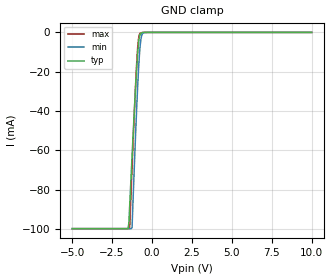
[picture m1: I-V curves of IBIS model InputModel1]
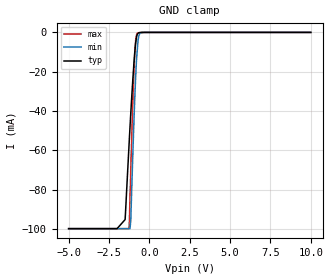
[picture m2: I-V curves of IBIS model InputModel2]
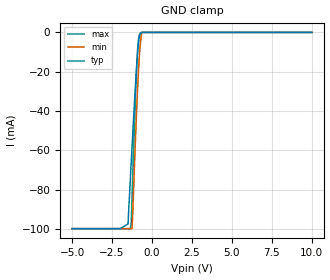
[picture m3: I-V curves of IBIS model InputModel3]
[IBIS Ver]   2.1
[File name]   e_200bx5.ibs   | e_= TSOP, f200bx= abbr chip name, 5= 5V Vcc
[File Rev]   2.00
[Date]   14-February-96
[Source]   File generated from lab measurements at Intel Corporation
[Notes]   Rev 2.00 All data was replaced by actual measurements
   performed in a lab.
[Disclaimer] INTEL DEVELOPER'S SOFTWARE LICENSE AGREEMENT
| BY USING THIS SOFTWARE, YOU ARE AGREEING TO BE BOUND
| BY THE TERMS OFTHIS AGREEMENT.  DO NOT USE THE SOFTWARE
| UNTIL YOU HAVE CAREFULLY READAND AGREED TO THE FOLLOWING
| TERMS AND CONDITIONS.  IF YOU DO NOT AGREETO THE TERMS
| OF THIS AGREEMENT, PROMPTLY RETURN THE SOFTWARE PACKAGE
| ANDANY ACCOMPANYING ITEMS.
| IF YOU USE THIS SOFTWARE, YOU WILL BE BOUND BY THE TERMS
| OF THIS AGREEMENT
| LICENSE: Intel Corporation ("Intel") grants you the non-exclusive right
| to use the enclosed software program ("Software").  You will not use,
| copy, modify, rent, sell or transfer the Software or any portion
| thereof, except as provided in this Agreement.
| System OEM Developers may:
| 1.   Copy the Software for support, backup or archival purposes;
| 2.   Install, use, or distribute Intel owned Software in object code
|   only;
| 3.   Modify and/or use Software source code that Intel directly makes
|   available to you as an OEM Developer;
| 4.   Install, use, modify, distribute, and/or make or have made
|   derivatives ("Derivatives") of Intel owned Software under the
|   terms and conditions in this Agreement, ONLY if you are a System
|   OEM Developer and NOT an end-user.
| RESTRICTIONS:
| YOU WILL NOT:
| 1.   Copy the Software, in whole or in part, except as provided for
|   in this Agreement;
| 2.   Decompile or reverse engineer any Software provided in object
|   code format;
| 3.   Distribute any Software or Derivative code to any end-users,
|   unless approved by Intel in a prior writing.
| TRANSFER: You may transfer the Software to another OEM
| Developer if thereceiving party agrees to the terms of this
| Agreement at the sole risk of any receiving party.
| OWNERSHIP AND COPYRIGHT OF SOFTWARE:
| Title to the Software and all copies thereof remain with Intel
| or its vendors.  The Software iscopyrighted and is protected by
| United States and international copyright laws.  You will not
| remove the copyright notice from the Software.  You agree to
| prevent any unauthorized copying of the Software.
| DERIVATIVE WORK: OEM Developers that make or have made
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[Copyright]   Copyright 1996, Intel Corporation, All Rights Reserved
[Component]   E28F200BX   | 56-lead TSOP package, 28F200BX
[Manufacturer]  Intel   | Boot Block (tm)
|   | operating in 5V Vcc range
[Package]
| Variable   typ   min   max
|The following values apply for the Copper leadframe.
R_pkg   48m   41m   54m
L_pkg   4.92nH   4.44nH   5.39nH
C_pkg   0.48pF   0.45pF   0.50pF
|The following values apply for the Alloy-42 leadframe.
|R_pkg   195m   180m   210m
|L_pkg   4.92nH   4.44nH   5.39nH
|C_pkg   0.48pF   0.45pF   0.50pF
|*****************************Pin Definitions**********************************
[Pin]   signal_name   model_name   R_pin   L_pin   C_pin
 1   NC   InputModel6
 2   NC   InputModel6
 3   A15   InputModel1
 4   A14   InputModel1
 5   A13   InputModel1
 6   A12   InputModel1
 7   A11   InputModel1
 8   A10   InputModel1
 9   A09   InputModel1
10   A08   InputModel1
11   NC   InputModel6
12   NC   InputModel6
13   WE#   InputModel5
14   RP#   InputModel3
15   NC   InputModel6
16   NC   InputModel6
17   VPP   POWER
18   DU   InputModel6
19   NC   InputModel6
20   NC   InputModel1
21   A07   InputModel1
22   A06   InputModel1
23   A05   InputModel1
24   A04   InputModel1
25   A03   InputModel1
26   A02   InputModel1
27   A01   InputModel1
28   NC   InputModel6
29   NC   InputModel6
30   NC   InputModel6
31   A0   InputModel2
32   CE#   InputModel2
33   GND   GND
34   OE#   InputModel4
35   DQ0   InputOutput1
36   DQ8   InputOutput1
37   DQ1   InputOutput1
38   DQ9   InputOutput1
39   DQ2   InputOutput1
40   DQ10   InputOutput1
41   DQ3   InputOutput1
42   DQ11   InputOutput1
43   VCC   POWER
44   VCC   POWER
45   DQ4   InputOutput1
46   DQ12   InputOutput1
47   DQ5   InputOutput1
48   DQ13   InputOutput1
49   DQ6   InputOutput1
50   DQ14   InputOutput1
51   DQ7   InputOutput1
52   DQ15   InputOutput2
53   GND   GND
54   BYTE#   InputModel2
55   A16   InputModel2
56   NC   InputModel6
|***********************Input Model 6******************************
[Model]   InputModel6
Model_type   Input
|   Model for DU and NC pins, excluding Pin #20.
Vinl = 0.8V
Vinh = 2.0V
|Variable   Typ   Min   Max
C_comp   5.61p   NA   7.6p
[Voltage Range]   5.0V   4.5V   5.5V
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| Models and submodels in the file (8): InputModel1 (Input), InputModel2 (Input), InputModel3 (Input), InputModel4 (Input), InputModel5 (Input), InputModel6 (Input), InputOutput1 (I/O), InputOutput2 (I/O)
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|*********************Input Model 1************************************
[Model]   InputModel1
Model_type   Input
|   Model for A[15:1] & NC (pin 20).
Vinl = 0.8V
Vinh = 2.0V
|Variable   Typ   Min   Max
C_comp   5.61p   NA   7.6p
[Voltage Range]   5.0V   4.5V   5.5V
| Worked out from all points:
|   GND clamp passes 1 mA (typ) near -0.75 V on its own axis
[GND_clamp]
|Voltage  I(typ)   I(min)   I(max)
-5V       -99.84mA   -99.85mA   -99.85mA
-1.5V     -99.84mA   -99.85mA   -99.85mA
-1.45V    -97.1mA    -99.85mA   -99.85mA
-1.4V     -88.66mA   -99.85mA   -99.85mA
-1.25V    -63.24mA   -99.36mA   -69.05mA
-1.05V    -31.09mA   -56.35mA   -30.63mA
-950mV    -16.83mA   -36.7mA    -14.35mA
-850mV    -5.99mA    -19.86mA   -3.6mA
-750mV    -1.015mA   -7.435mA   -471.4uA
-650mV    -202.7uA   -1.654mA   -140.8uA
-500mV    -27.26uA   -101.4uA   -12.27uA
10V       0A         0A         0A
[Power_clamp]
| Input buffer circuits of this product do not intrinsically
| require a [Power_clamp] definition.  This zero current
| [Power_clamp] table is provided for the compatibility with
| some IBIS parsers.
|Voltage  I(typ)   I(min)   I(max)
-5V       0A         0A         0A
0V        0A         0A         0A
5V        0A         0A         0A
10V       0A         0A         0A
|*********************Input Model 2******************************
[Model]   InputModel2
Model_type   Input
|   Model for A[0], A[16], CE# & BYTE# pins.
Vinl = 0.8V
Vinh = 2.0V
|Variable   Typ   Min   Max
C_comp   5.61p   NA   7.6p
[Voltage Range]   5.0V   4.5V   5.5V
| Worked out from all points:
|   GND clamp passes 1 mA (typ) near -0.75 V on its own axis
[GND_clamp]
|Voltage  I(typ)   I(min)   I(max)
-5V       -99.84mA   -99.85mA   -99.85mA
-2V       -99.84mA   -99.85mA   -99.85mA
-1.5V     -95.21mA   -99.85mA   -99.85mA
-1.25V    -55.95mA   -99.85mA   -99.68mA
-1.2V     -48.44mA   -99.85mA   -84.47mA
-1.15V    -41.14mA   -95.68mA   -69.64mA
-950mV    -15.15mA   -43.95mA   -18.45mA
-850mV    -5.666mA   -23.02mA   -4.089mA
-750mV    -1.032mA   -9.168mA   -475.6uA
-650mV    -207.5uA   -1.728mA   -133.8uA
-500mV    -28.64uA   -98.99uA   -10.29uA
10V       0A         0A         0A
[Power_clamp]
| Input buffer circuits of this product do not intrinsically
| require a [Power_clamp] definition.  This zero current
| [Power_clamp] table is provided for the compatibility with
| some IBIS parsers.
|Voltage  I(typ)   I(min)   I(max)
-5V       0A         0A         0A
0V        0A         0A         0A
5V        0A         0A         0A
10V       0A         0A         0A
|***********************Input Model 3******************************
[Model]   InputModel3
Model_type   Input
|   Model for RP# pin.
Vinl = 0.8V
Vinh = 2.0V
|Variable   Typ   Min   Max
C_comp   5.61p   NA   7.6p
[Voltage Range]   5.0V   4.5V   5.5V
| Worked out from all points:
|   GND clamp passes 1 mA (typ) near -0.75 V on its own axis
[GND_clamp]
|Voltage  I(typ)   I(min)   I(max)
-5V       -99.85mA   -99.85mA   -99.85mA
-2V       -99.85mA   -99.85mA   -99.85mA
-1.5V     -97.47mA   -99.85mA   -99.85mA
-1.35V    -73.75mA   -99.85mA   -99.85mA
-1.3V     -65.95mA   -99.85mA   -96.97mA
-1.25V    -58.19mA   -99.85mA   -83.97mA
-1.05V    -28.67mA   -57.7mA    -35.89mA
-950mV    -15.59mA   -37.45mA   -16.08mA
-850mV    -5.621mA   -20.13mA   -3.693mA
-750mV    -981uA     -7.476mA   -460uA
-650mV    0A         0A         0A
10V       0A         0A         0A
[Power_clamp]
| Input buffer circuits of this product do not intrinsically
| require a [Power_clamp] definition.  This zero current
| [Power_clamp] table is provided for the compatibility with
| some IBIS parsers.
|Voltage  I(typ)   I(min)   I(max)
-5V       0A         0A         0A
0V        0A         0A         0A
5V        0A         0A         0A
10V       0A         0A         0A
